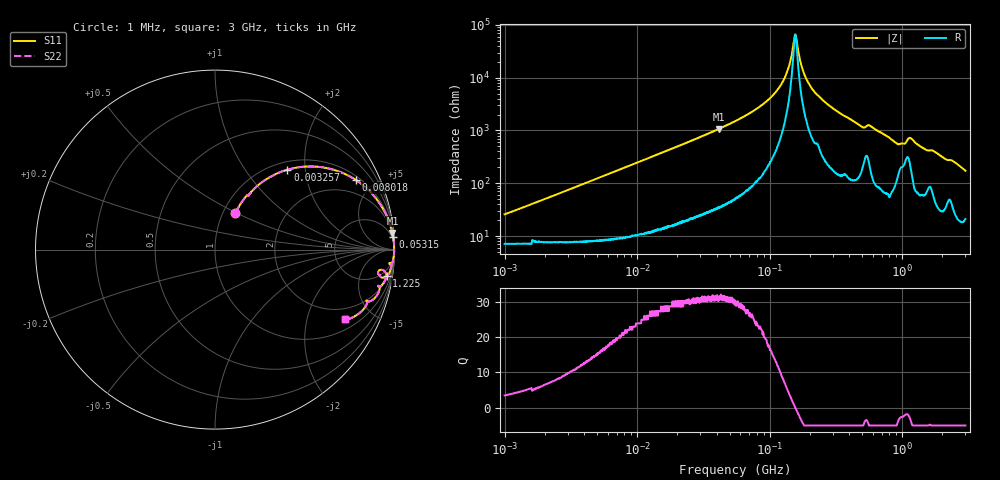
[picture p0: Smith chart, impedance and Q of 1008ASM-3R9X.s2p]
!s-Parameter Generated by FASTRON Sdn. Bhd.
!FASTRON P/N : 1008ASM-3R9X
!Keysight Technologies: E4991B_MY54100416_A.01.15
!Date: Wed Jun 19 15:38:38 2024
!Version  :Rev00  Wed Jun 19 15:38:38 2024
!Data & Calibration Information:
!Freq  S11  S21  S12  S22
!PortZ  Port1:50+j0  Port2:50+j0
!When reading reference impedance value at option line is always used.
! Remarks : This data is being provided solely for informational purposes.
# Hz S dB R 50
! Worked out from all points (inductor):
!   1601 points, 1 MHz to 3 GHz, reference 50 ohm
!   read as one part in series: L = 3.94 uH near 1.041 MHz
!   highest Q = 31.3 at 41.18 MHz (marker M1), where L = 4.11 uH
!   self-resonance near 155.9 MHz
!   S11 on the Smith chart (normalised r, x): 1 MHz: 1.14, +0.50; 3.257 MHz: 1.15, +1.61; 8.018 MHz: 1.18, +3.95; 53.15 MHz: 2, +29; 1.225 GHz: 3, -12; 3 GHz: 1.42, -3.43
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1000000  -12.60 61.0  -0.82 -13.0  -0.82 -13.0  -12.60 61.0
3257432  -4.43 47.8  -2.56 -36.7  -2.56 -36.7  -4.43 47.8
3804036  -3.63 44.2  -3.10 -41.0  -3.10 -41.0  -3.63 44.2
8017732  -1.15 26.3  -7.06 -61.0  -7.06 -61.0  -1.15 26.3
1.447069e7  -0.41 15.5  -11.50 -72.4  -11.50 -72.4  -0.41 15.5
4.118017e7  -0.06 5.3  -20.60 -82.8  -20.60 -82.8  -0.06 5.3
5.315222e7  -0.04 4.0  -23.20 -84.1  -23.20 -84.1  -0.04 4.0
5.504702e7  -0.04 3.8  -23.60 -84.3  -23.60 -84.3  -0.04 3.8
8.636184e7  -0.02 1.9  -29.50 -85.5  -29.50 -85.5  -0.02 1.9
1.15443e8  -0.01 0.9  -35.70 -84.2  -35.70 -84.2  -0.01 0.9
1.361705e8  -0.01 0.4  -42.50 -78.5  -42.50 -78.5  -0.01 0.4
1.558689e8  -0.01 0.0  -56.40 -5.0  -56.40 -5.0  -0.01 0.0
1.606197e8  -0.01 -0.1  -53.50 44.0  -53.50 44.0  -0.01 -0.1
1.793119e8  -0.01 -0.4  -42.40 77.2  -42.40 77.2  -0.01 -0.4
2.083556e8  -0.02 -0.9  -35.90 82.5  -35.90 82.5  -0.02 -0.9
3.471137e8  -0.04 -2.8  -26.30 83.3  -26.30 83.3  -0.04 -2.8
7.925923e8  -0.17 -7.6  -17.60 78.0  -17.60 78.0  -0.17 -7.6
9.255909e8  -0.48 -9.6  -15.40 66.8  -15.40 66.8  -0.48 -9.6
1.136371e9  -0.47 -7.0  -17.70 62.5  -17.70 62.5  -0.47 -7.0
1.22495e9  -0.29 -8.8  -16.30 73.3  -16.30 73.3  -0.29 -8.8
1.912199e9  -0.56 -15.8  -11.30 69.0  -11.30 69.0  -0.56 -15.8
3e9  -1.69 -28.2  -6.45 54.8  -6.45 54.8  -1.69 -28.2
